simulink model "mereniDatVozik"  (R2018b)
settings: Solver=ode4  StartTime=0.0  StopTime=inf  FixedStep=1e-3  RelTol=1e-3
undefined symbols (not defined in the file or in its folder): Humusoft, MF624
libraries: sldrtlib x7, simulink x3, powerlib_meascontrol x1

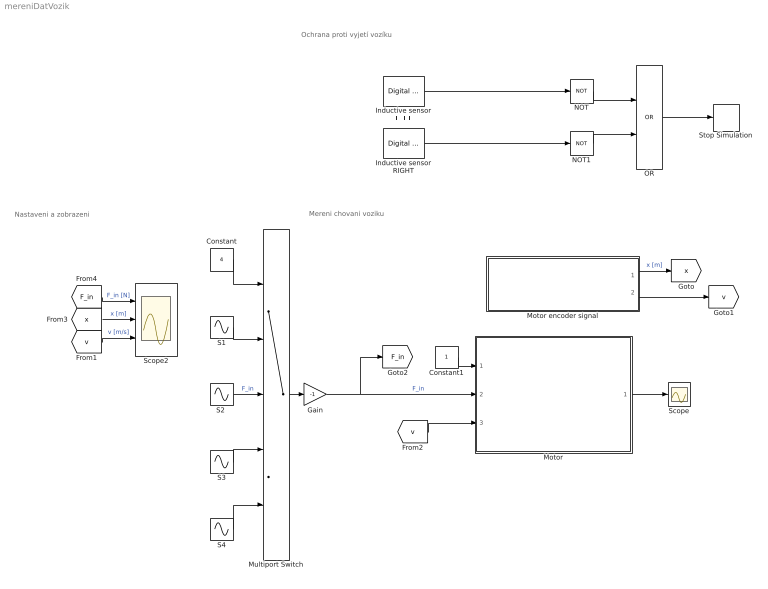
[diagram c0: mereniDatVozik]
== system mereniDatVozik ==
  note: Nastaveni a zobrazeni
  note: Mereni chovani voziku
  note: Ochrana proti vyjetí vozíku
  Constant : Constant  Value=4
  Constant1 : Constant
  Gain : Gain  Gain=-1
  Inductive sensor LEFT : sldrtlib/Digital Input  SampleTime=0.001  MaxMissedTicks=1e6  ShowMissedTicks=off  YieldWhenWaiting=off  DrvName=Humusoft/MF624  DrvAddress=4294967295  DrvOptions=0  Channels=1  BitMode=1  DataType=1
  Inductive sensor RIGHT : sldrtlib/Digital Input  SampleTime=0.001  MaxMissedTicks=1e6  ShowMissedTicks=off  YieldWhenWaiting=off  DrvName=Humusoft/MF624  DrvAddress=4294967295  DrvOptions=0  Channels=2  BitMode=1  DataType=1
  Motor : Subsystem
  Motor encoder signal : Subsystem
  Multiport Switch : MultiPortSwitch  Inputs=4
  NOT : Logic  Operator=NOT  IconShape=distinctive  AllPortsSameDT=off  OutDataTypeStr=boolean
  NOT1 : Logic  Operator=NOT  IconShape=distinctive  AllPortsSameDT=off  OutDataTypeStr=boolean
  OR : Logic  Operator=OR  IconShape=distinctive  AllPortsSameDT=off  OutDataTypeStr=boolean
  S1 : Sin  Amplitude=8  Frequency=1.5*pi  SampleTime=0
  "S2 " : Sin  Amplitude=10  Frequency=1.8*pi  SampleTime=0
  S3 : Sin  Amplitude=5  Frequency=1.4*pi  SampleTime=0
  S4 : Sin  Amplitude=4  Frequency=0.9*pi  SampleTime=0
  Scope : Scope
  Scope2 : Scope  NumInputPorts=3
  Stop Simulation : Stop
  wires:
  Motor encoder signal/2(v [m/s]) -> [v]
  Motor encoder signal/1(x [m]) -> [x]  "x [m]"
  Inductive sensor RIGHT/1 -> NOT1/1
  NOT1/1 -> OR/2
  NOT/1 -> OR/1
  Inductive sensor LEFT/1 -> NOT/1
  OR/1 -> Stop Simulation/1
  [v] -> Motor/3(v [m/s])
  Motor/1(sat_flag) -> Scope/1
  [x] -> Scope2/2  "x [m]"
  [F_in] -> Scope2/1  "F_in [N]"
  [v] -> Scope2/3  "v [m/s]"
  Multiport Switch/1 -> Gain/1
  Constant/1 -> Multiport Switch/1
  S1/1 -> Multiport Switch/2
  S3/1 -> Multiport Switch/4
  S4/1 -> Multiport Switch/5
  Constant1/1 -> Motor/1(ENABLE)
  Gain/1 -> [F_in], Motor/2(F_in [N])  "F_in"
  "S2 "/1 -> Multiport Switch/3  "F_in"

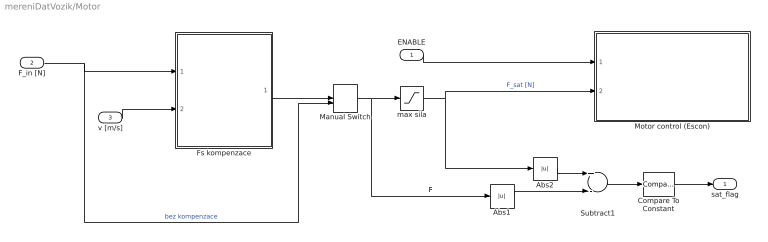
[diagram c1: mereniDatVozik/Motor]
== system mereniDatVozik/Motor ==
  ENABLE : Inport
  F_in [N] : Inport  Port=2
  v [m/s] : Inport  Port=3
  Abs1 : Abs
  Abs2 : Abs
  Compare To Constant : simulink/Logic and Bit Operations/Compare To Constant  relop=>  const=1e-8  OutDataTypeStr=boolean
  Fs kompenzace : Subsystem
  Manual Switch : ManualSwitch
  Motor control (Escon) : Subsystem
  Subtract1 : Sum  Inputs=+-
  max sila : Saturate  UpperLimit=40  LowerLimit=-40
  sat_flag : Outport
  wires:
  ENABLE/1 -> Motor control (Escon)/1(ENABLE)
  v [m/s]/1 -> Fs kompenzace/2(v [m/s])
  F_in [N]/1 -> Fs kompenzace/1(F_in [N]), Manual Switch/2  "bez kompenzace"
  Fs kompenzace/1(F_out [N]1) -> Manual Switch/1
  Abs2/1 -> Subtract1/1
  Manual Switch/1 -> Abs1/1, max sila/1  "F"
  Subtract1/1 -> Compare To Constant/1
  Abs1/1 -> Subtract1/2
  max sila/1 -> Abs2/1, Motor control (Escon)/2(Ref strength [N])  "F_sat [N]"
  Compare To Constant/1 -> sat_flag/1

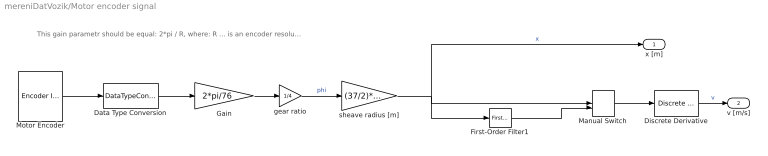
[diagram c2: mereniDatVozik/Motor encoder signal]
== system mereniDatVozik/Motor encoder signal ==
  note: This gain parametr should be equal: 2*pi / R, where: R ... is an encoder resolution
  Data Type Conversion : DataTypeConversion  OutDataTypeStr=double
  Discrete Derivative : simulink/Discrete/Discrete Derivative  gainval=1.0  ICPrevScaledInput=0.0  OutMin=[]  OutMax=[]  OutDataType=fixdt(1, 16)  OutScaling=2^-10  DoSatur=off
  First-Order Filter1 : powerlib_meascontrol/Filters/First-Order Filter  FilterType=Lowpass  Tc=0.004  Ts=0.001  Initialize=on  Vac_Init=[0, 0, 60]  Vdc_Init=0  PlotResponse=off  FreqRange="[0,  200,  1]"
  Gain : Gain  Gain=2*pi/76
  Manual Switch : ManualSwitch  CurrentSetting=0
  Motor Encoder : sldrtlib/Encoder Input  SampleTime=0.001  MaxMissedTicks=1e8  ShowMissedTicks=off  YieldWhenWaiting=off  DrvName=Humusoft/MF624  DrvAddress=4294967295  DrvOptions=0  Channels=3  QuadMode=3  IndexPulse=1  InputFilter=Inf  DataType=7
  gear ratio : Gain  Gain=1/4
  sheave radius [m] : Gain  Gain=(37/2)*1e-3
  x [m] : Outport
  v [m/s] : Outport  Port=2
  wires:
  Motor Encoder/1 -> Data Type Conversion/1
  Discrete Derivative/1 -> v [m/s]/1  "v"
  Data Type Conversion/1 -> Gain/1
  Gain/1 -> gear ratio/1
  sheave radius [m]/1 -> First-Order Filter1/1, Manual Switch/1, x [m]/1  "x"
  gear ratio/1 -> sheave radius [m]/1  "phi"
  First-Order Filter1/1 -> Manual Switch/2
  Manual Switch/1 -> Discrete Derivative/1

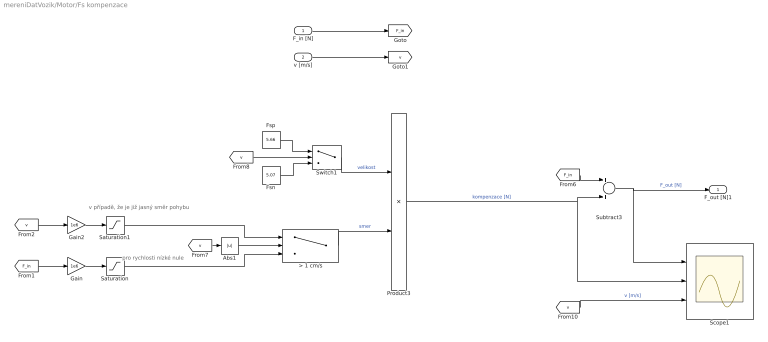
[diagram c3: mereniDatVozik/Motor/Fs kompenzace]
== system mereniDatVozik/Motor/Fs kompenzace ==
  note: v případě, že je již jasný směr pohybu
  note: pro rychlosti nízké nule
  F_in [N] : Inport
  v [m/s] : Inport  Port=2
  > 1 cm/s : Switch  Threshold=1e-2
  Abs1 : Abs
  Fsn : Constant  Value=5.07
  Fsp : Constant  Value=5.66
  Gain : Gain  Gain=1e6
  Gain2 : Gain  Gain=1e6
  Product3 : Product
  Saturation : Saturate  UpperLimit=1  LowerLimit=-1
  Saturation1 : Saturate  UpperLimit=1  LowerLimit=-1
  Scope1 : Scope  NumInputPorts=3
  Subtract3 : Sum
  Switch1 : Switch
  F_out [N]1 : Outport
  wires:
  F_in [N]/1 -> [F_in]
  v [m/s]/1 -> [v]
  Fsn/1 -> Switch1/3
  [v] -> Switch1/2
  Fsp/1 -> Switch1/1
  [F_in] -> Subtract3/1
  [v] -> Scope1/3  "v [m/s]"
  Subtract3/1 -> F_out [N]1/1, Scope1/1  "F_out [N]"
  Switch1/1 -> Product3/1  "velikost"
  > 1 cm/s/1 -> Product3/2  "smer"
  Product3/1 -> Subtract3/2, Scope1/2  "kompenzace [N]"
  Saturation/1 -> > 1 cm/s/3
  Saturation1/1 -> > 1 cm/s/1
  [v] -> Gain2/1
  Abs1/1 -> > 1 cm/s/2
  [F_in] -> Gain/1
  Gain/1 -> Saturation/1
  [v] -> Abs1/1
  Gain2/1 -> Saturation1/1

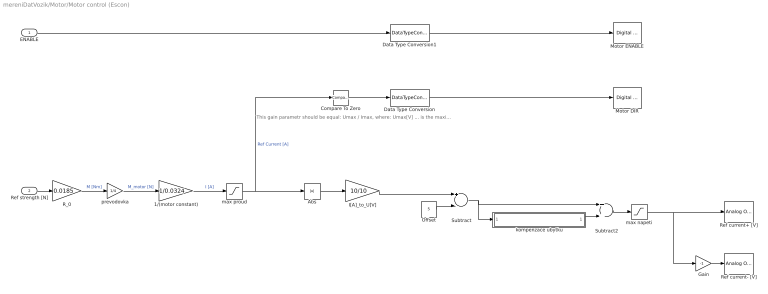
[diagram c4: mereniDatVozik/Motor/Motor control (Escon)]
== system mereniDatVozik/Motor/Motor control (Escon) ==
  note: This gain parametr should be equal: Umax / Imax, where: Umax[V] ... is the maximum absolute value of the output voltage (for MF624 Umax = 10 V ... think about MF624 isolation board voltage reduction ) Imax[A] ... is the maximum allowed current
  ENABLE : Inport
  Ref strength [N] : Inport  Port=2
  1/(motor constant) : Gain  Gain=1/0.0324
  Abs : Abs
  Compare To Zero : simulink/Logic and Bit Operations/Compare To Zero  relop=>=  OutDataTypeStr=boolean
  Data Type Conversion : DataTypeConversion  OutDataTypeStr=boolean
  Data Type Conversion1 : DataTypeConversion  OutDataTypeStr=boolean
  Gain : Gain  Gain=-1
  I[A]_to_U[V] : Gain  Gain=10/10
  Motor DIR : sldrtlib/Digital Output  SampleTime=0.001  MaxMissedTicks=1e6  ShowMissedTicks=off  YieldWhenWaiting=off  DrvName=Humusoft/MF624  DrvAddress=4294967295  DrvOptions=0  Channels=5  BitMode=1  InitialValue=[]  FinalValue=[]
  Motor ENABLE : sldrtlib/Digital Output  SampleTime=0.001  MaxMissedTicks=1e6  ShowMissedTicks=off  YieldWhenWaiting=off  DrvName=Humusoft/MF624  DrvAddress=4294967295  DrvOptions=0  Channels=2  BitMode=1  InitialValue=0  FinalValue=0
  Offset : Constant  Value=5
  R_0 : Gain  Gain=0.0185
  Ref current+ [V] : sldrtlib/Analog Output  SampleTime=0.001  MaxMissedTicks=1e6  ShowMissedTicks=off  YieldWhenWaiting=off  DrvName=Humusoft/MF624  DrvAddress=4294967295  DrvOptions=0  Channels=6  RangeMode=1  VoltRange=1  InitialValue=-5  FinalValue=-5
  Ref current- [V] : sldrtlib/Analog Output  SampleTime=0.001  MaxMissedTicks=1e6  ShowMissedTicks=off  YieldWhenWaiting=off  DrvName=Humusoft/MF624  DrvAddress=4294967295  DrvOptions=0  Channels=5  RangeMode=1  VoltRange=1  InitialValue=5  FinalValue=5
  Subtract : Sum  Inputs=+-
  Subtract2 : Sum
  kompenzace ubytku : Subsystem
  max napeti : Saturate  UpperLimit=5.5  LowerLimit=-5.5
  max proud : Saturate  UpperLimit=10  LowerLimit=-10
  prevodovka : Gain  Gain=1/4
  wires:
  Data Type Conversion/1 -> Motor DIR/1
  Abs/1 -> I[A]_to_U[V]/1
  Gain/1 -> Ref current- [V]/1
  Compare To Zero/1 -> Data Type Conversion/1
  Data Type Conversion1/1 -> Motor ENABLE/1
  I[A]_to_U[V]/1 -> Subtract/1
  1/(motor constant)/1 -> max proud/1  "I [A]"
  max proud/1 -> Abs/1, Compare To Zero/1  "Ref Current [A]"
  Ref strength [N]/1 -> R_0/1
  max napeti/1 -> Gain/1, Ref current+ [V]/1
  Offset/1 -> Subtract/2
  ENABLE/1 -> Data Type Conversion1/1
  Subtract2/1 -> max napeti/1
  kompenzace ubytku/1(error compensation [V]) -> Subtract2/2
  Subtract/1 -> kompenzace ubytku/1(voltage out [V]), Subtract2/1
  R_0/1 -> prevodovka/1  "M [Nm]"
  prevodovka/1 -> 1/(motor constant)/1  "M_motor [N]"

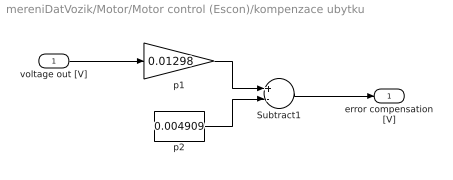
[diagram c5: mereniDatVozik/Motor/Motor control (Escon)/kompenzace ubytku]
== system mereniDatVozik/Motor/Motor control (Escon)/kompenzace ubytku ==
  voltage out [V] : Inport
  Subtract1 : Sum  Inputs=+-
  p1 : Gain  Gain=0.01298
  p2 : Constant  Value=0.004909
  error compensation [V] : Outport
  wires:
  p1/1 -> Subtract1/1
  p2/1 -> Subtract1/2
  Subtract1/1 -> error compensation [V]/1
  voltage out [V]/1 -> p1/1
